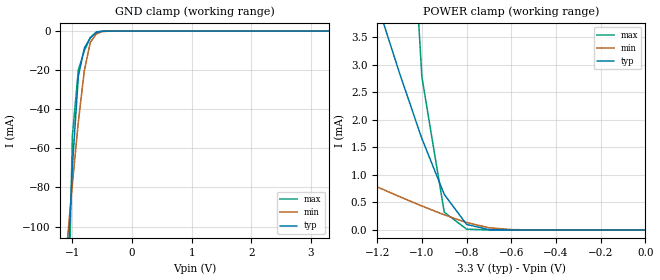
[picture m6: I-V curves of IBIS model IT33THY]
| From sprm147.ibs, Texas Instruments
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[Model]   IT33THY
Model_type   Input
Polarity   Non-Inverting
| signals   A, Y
Vinl = 0.8V
Vinh = 2.0V
|   typ   min   max
C_comp   0.8606482p   0.83185155p   0.89077786p
|   typ   min   max
[Temperature Range]   25   -40   125
|   typ   min   max
[Voltage Range]   3.30V   3.00V   3.60V
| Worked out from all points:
|   GND clamp passes 1 mA (typ) near -0.61 V on its own axis
|   POWER clamp passes 1 mA (typ) near -0.93 V on its own axis
[GND_clamp]
|   Voltage   I(typ)   I(min)   I(max)
-3.3V     -1.924A    -954.8mA   -4.929A
-1.1V     -136mA     -112.6mA   -192.1mA
-1V       -69.42mA   -78.28mA   -53.73mA
-900mV    -23.15mA   -46.5mA    -19.88mA
-800mV    -8.734mA   -20.34mA   -10.13mA
-700mV    -3.437mA   -5.821mA   -3.396mA
-600mV    -755.6uA   -1.469mA   -483.1uA
-500mV    -77.66uA   -274uA     -28.67uA
-400mV    -4.875uA   -34.93uA   -866.3nA
3.3V      177.6pA    11.68nA    0A
[POWER_clamp]
|   Voltage   I(typ)   I(min)   I(max)
-3.3V     33.03mA    4.773mA    224.5mA
-2.7V     24.64mA    3.607mA    164.7mA
-1.8V     12.17mA    1.89mA     75.57mA
-1.2V     4.113mA    781.6uA    18.29mA
-1.1V     2.848mA    605.4uA    9.702mA
-1V       1.658mA    435uA      2.778mA
-900mV    646uA      274.8uA    323.3uA
-800mV    100.4uA    135.2uA    14.29uA
-700mV    6.235uA    40.32uA    116.8nA
-600mV    176.8nA    6.906uA    888.2pA
-500mV    5.063nA    714.3nA    88.82pA
0V        1pA        1pA        1pA
